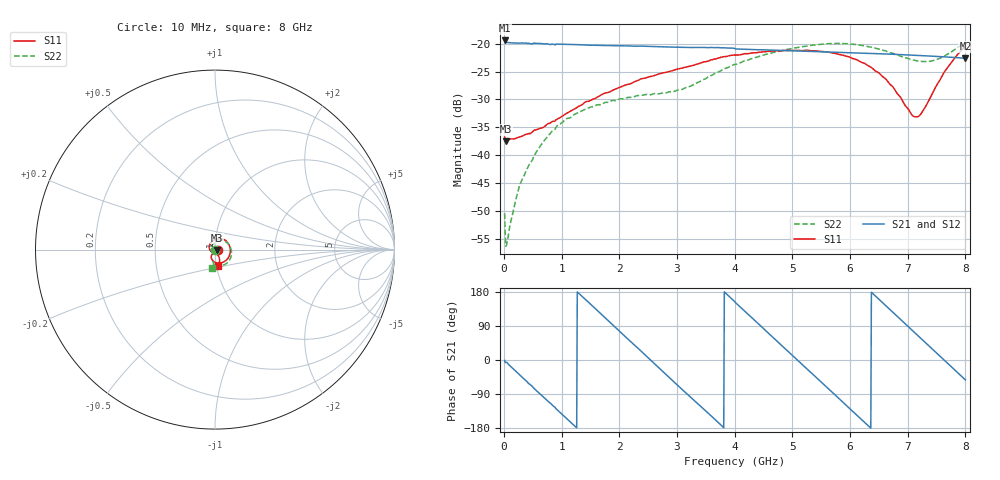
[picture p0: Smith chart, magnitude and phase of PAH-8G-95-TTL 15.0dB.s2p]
! MTS Systemtechnik GmbH
! S-Parameters
! Model: PAH-8G/95-TTL
! Attenuation Step: 15.0dB
! Rohde & Schwarz ZVB8 2Ports - Version 4.11 - 1145.1010k08 SN: 100119
! S2P File Measurements:
! S11 S21 S12 S22
# HZ  S  DB  R  50.00
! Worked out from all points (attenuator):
!   800 points, 10 MHz to 8 GHz, reference 50 ohm
!   highest |S21| = -19.43 dB at 10 MHz (marker M1); lowest = -22.6 dB at 8 GHz (marker M2)
!   lowest |S11| = -37.5 dB at 30 MHz (marker M3), VSWR 1.03, Z = 51.3 - j0.217 ohm
!   |S11| at or under -10 dB: start of sweep to end of sweep
!   |S22| runs from -56.3 to -19.8 dB; largest |S21 - S12| = 0.0016
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1e7  -36.74 -10.3  -19.43 -1.2  -19.34 -1.1  -50.39 -85.6
3e7  -37.50 -9.1  -19.84 -6.4  -19.86 -6.4  -56.27 -97.9
7e7  -37.25 -11.6  -19.81 -10.2  -19.82 -10.2  -54.69 -90.9
2.7e8  -36.71 -41.4  -19.91 -39.1  -19.92 -39.1  -45.43 -110.7
5.6e8  -35.41 -83.9  -19.95 -80.7  -19.98 -80.5  -39.39 -139.3
9.4e8  -33.42 -133.8  -20.10 -133.9  -20.09 -134.0  -34.54 -171.8
1.35e9  -30.96 -176.9  -20.22 168.2  -20.23 168.2  -32.03 156.7
1.96e9  -28.03 137.2  -20.39 81.5  -20.40 81.6  -30.15 117.8
2.68e9  -25.45 97.1  -20.55 -19.9  -20.55 -19.7  -28.98 90.6
3.28e9  -23.89 68.8  -20.69 -104.4  -20.71 -104.8  -27.35 75.6
3.68e9  -22.73 51.1  -20.71 -160.1  -20.68 -159.6  -25.18 64.3
4.01e9  -22.08 33.7  -20.96 151.8  -20.95 151.7  -23.77 49.9
4.57e9  -21.39 4.2  -21.14 72.8  -21.15 72.8  -21.88 22.7
4.97e9  -21.23 -18.2  -21.27 16.3  -21.28 16.1  -20.93 0.8
5.34e9  -21.29 -39.5  -21.40 -35.7  -21.42 -35.7  -20.30 -19.6
5.72e9  -21.72 -62.4  -21.53 -89.2  -21.56 -89.3  -19.99 -41.2
6.11e9  -22.86 -87.5  -21.67 -144.5  -21.69 -144.6  -20.18 -63.2
6.67e9  -27.00 -118.0  -21.87 136.3  -21.89 136.3  -21.56 -89.8
7.07e9  -32.76 -104.8  -22.07 79.5  -22.07 79.4  -22.89 -99.0
7.18e9  -33.06 -87.3  -22.12 63.8  -22.13 63.8  -23.17 -98.8
7.65e9  -24.86 -63.7  -22.38 -2.7  -22.39 -2.8  -22.14 -94.6
8e9  -20.47 -80.0  -22.63 -52.4  -22.63 -52.4  -19.76 -98.9
